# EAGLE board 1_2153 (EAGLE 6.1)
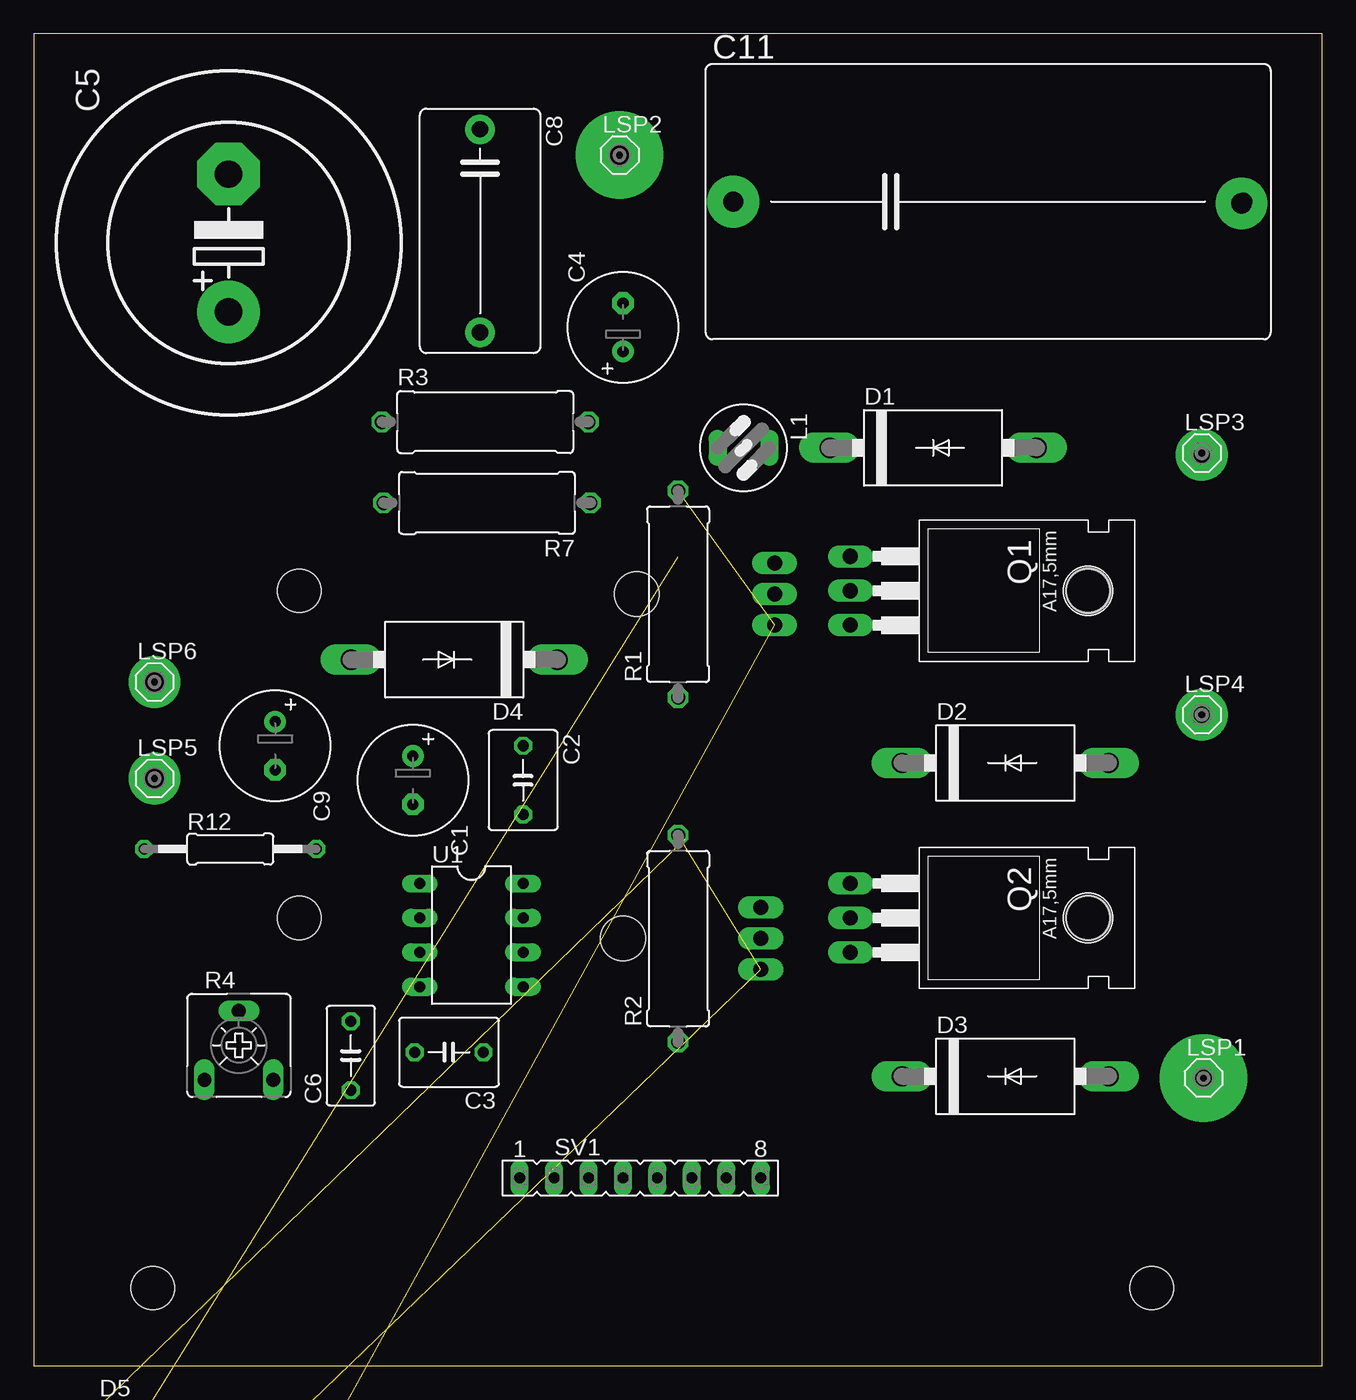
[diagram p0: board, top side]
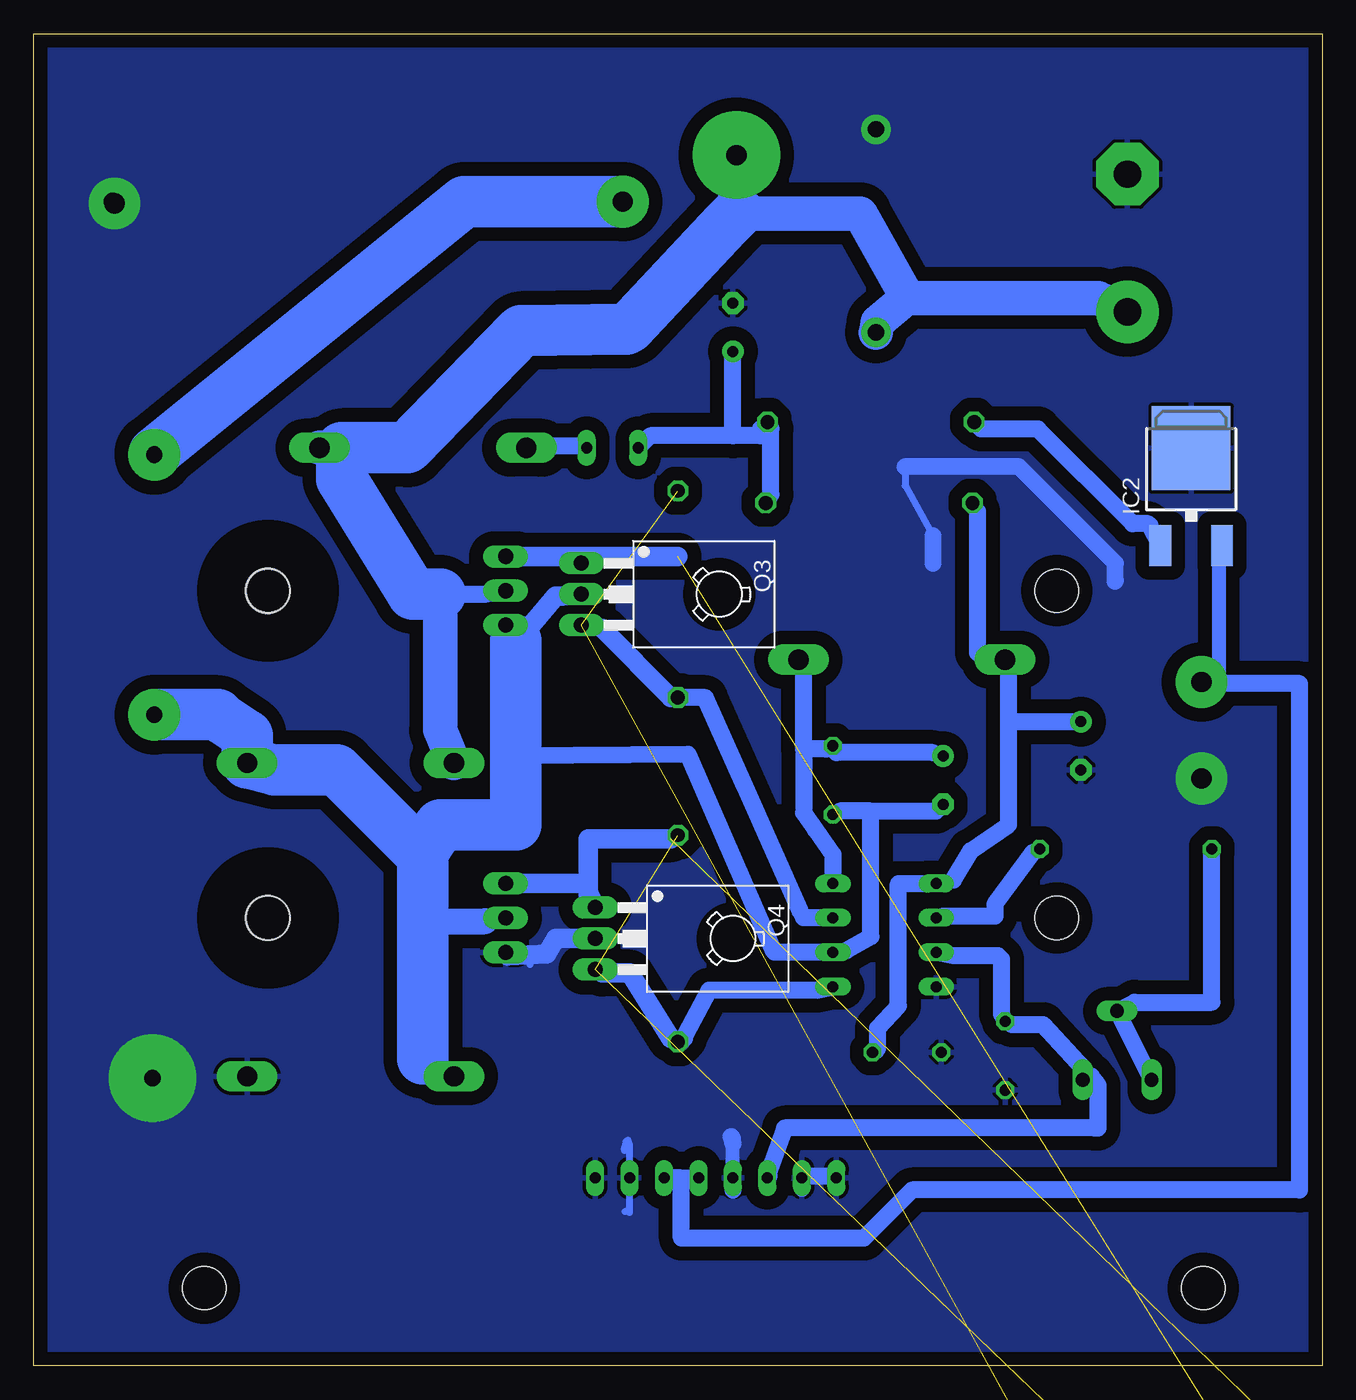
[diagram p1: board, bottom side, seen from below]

Size 94.98 x 98.22 mm. Coordinates in mm from the lower left corner, seen from the top.
Outline: 0,0 94.98,0 94.98,98.22 0,98.22 0,0
Copper layers (1*16): Top 0.035mm / dielectric 1.5mm / Bottom 0.035mm
Design rules: minimum track width 20mil, minimum drill 24mil, track to track 10mil, track to pad 15mil, pad to pad 8mil, via to via 8mil, smd to smd 8mil, copper to edge 40mil, drill to drill 8mil, minimum pad ring 10mil, minimum via ring 8mil, stop-mask expansion 4mil, vias tented up to drill 0mil, thermal gap 10mil
Holes 3.2 mm at 19.56,57.15 19.56,33.02 8.76,5.71 82.42,5.71 77.72,57.15 77.72,33.02

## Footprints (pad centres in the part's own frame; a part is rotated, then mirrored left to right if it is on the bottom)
E3,5-8 = drill 0.813 pad 1.6: + -1.778,0 | drill 0.813 pad 1.6 octagon: - 1.778,0
C050-050X075 = drill 0.813 octagon: 1 -2.54,0; 2 2.54,0
EB25D = drill 2.007 pad 4.597: + -5.08,0 | drill 2.007 pad 4.597 octagon: - 5.08,0
C050-035X075 = drill 0.813 octagon: 1 -2.54,0; 2 2.54,0
C150-091X182 = drill 1.016 octagon: 1 -7.493,0; 2 7.493,0
C375-203X418 = drill 1.321 octagon: 1 -18.796,0; 2 18.796,0
DO201-15 = drill 1.499 long: A 7.62,0; C -7.62,0
DPACK = smd 1.6 x 3: 1 -2.28,-4.8; 3 2.28,-4.8 | smd 5.8 x 6.2: 4 0,2.38
82114R = drill 0.813 long: 1 0,1.905; 2 0,-1.905
MCS10B = drill 1.016 pad 2.159 octagon: MP 0,0
TO220 = drill 1.118 long: 1 -2.54,-6.35; 2 0,-6.35; 3 2.54,-6.35 | hole 3.302: 0,11.176
TO126 = drill 1.118 long: 1 -2.286,-5.08; 2 0,-5.08; 3 2.286,-5.08 | hole 3.302: 0,5.08
P0613/15 = drill 1.016 octagon: 1 -7.62,0; 2 7.62,0
CA6V = drill 1.016 long: A -2.54,-2.54; E 2.54,-2.54; S 0,2.54
0207/12 = drill 0.813 octagon: 1 -6.35,0; 2 6.35,0
FE08 = drill 0.813 long: 1 -8.89,0; 2 -6.35,0; 3 -3.81,0; 4 -1.27,0; 5 1.27,0; 6 3.81,0; 7 6.35,0; 8 8.89,0
DIL08 = drill 0.813 long: 1 -3.81,-3.81; 2 -1.27,-3.81; 3 1.27,-3.81; 4 3.81,-3.81; 5 3.81,3.81; 6 1.27,3.81; 7 -1.27,3.81; 8 -3.81,3.81

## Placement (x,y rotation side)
C1  100x16  [E3,5-8]  27.94,43.18 270 top
C2  0.33  [C050-050X075]  36.07,43.18 270 top
C3  0.33  [C050-050X075]  30.61,23.11 180 top
C4  100x16  [E3,5-8]  43.43,76.58 90 top
C5  [EB25D]  14.35,82.8 90 top
C6  2.2n  [C050-035X075]  23.37,22.86 90 top
C8  2.0  [C150-091X182]  32.89,83.69 270 top
C9  100x35  [E3,5-8]  17.78,45.72 270 top
C11  [C375-203X418]  70.36,85.85 0 top
D1  1N5400  [DO201-15]  66.29,67.69 0 top
D2  1N5400  [DO201-15]  71.63,44.45 0 top
D3  1N5400  [DO201-15]  71.63,21.34 0 top
D4  1N5400  [DO201-15]  30.99,52.07 180 top
D5  1N5400  [DO201-15]  not placed on the board
D6  1N5400  [DO201-15]  not placed on the board
IC2  7812  [DPACK]  9.65,65.28 0 bottom
L1  100mkGn  [82114R]  52.32,67.69 270 top
LSP1  MCS10B  [MCS10B]  86.23,21.21 0 top
LSP2  MCS10B  [MCS10B]  43.18,89.28 0 top
LSP3  MCS10B  [MCS10B]  86.11,67.31 0 top
LSP4  MCS10B  [MCS10B]  86.11,48.01 0 top
LSP5  MCS10B  [MCS10B]  8.89,43.31 0 top
LSP6  MCS10B  [MCS10B]  8.89,50.42 0 top
Q1  IRL3705  [TO220]  66.55,57.15 270 top
Q2  IRL3705  [TO220]  66.55,33.02 270 top
Q3  [TO126]  49.53,56.9 270 bottom
Q4  BD140  [TO126]  48.51,31.5 270 bottom
R1  100  [P0613/15]  47.5,56.9 90 top
R2  100  [P0613/15]  47.5,31.5 90 top
R3  100E  [P0613/15]  33.27,69.6 0 top
R4  10k  [CA6V]  15.11,23.62 0 top
R7  240E  [P0613/15]  33.4,63.63 180 top
R12  1k  [0207/12]  14.48,38.1 0 top
SV1  [FE08]  44.7,13.84 0 top
U1  IR2153  [DIL08]  32.26,31.75 270 top

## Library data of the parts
C1-C6 C8 C9 C11 R1-R3 R7 R12 = rcl
D1-D6 = diode
IC2 = v-reg
L1 = inductors
LSP1-LSP6 = solpad
Q1 Q2 = transistor-fet
Q3 Q4 = transistor-pnp
R4 = pot
SV1 = con-lsta
U1 = irf

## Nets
COM: C6.2 R4.E SV1.3 U1.3
GND: C3.2 C4.- C5.- C6.1 C8.1 C9.- C11.2 D3.A IC2.4 LSP1.MP LSP5.MP Q2.3 Q4.2 SV1.1 SV1.2 SV1.4 SV1.7 SV1.8 U1.4
N$1: D6.A Q3.3 R1.2
N$2: R12.2 U1.2
N$3: D5.A Q4.3 R2.2
N$4: C4.+ L1.2 R3.2 R7.1
N$5: R1.1 U1.7
N$6: R4.A R4.S R12.1
N$7: IC2.3 LSP6.MP SV1.5 SV1.6
N$8: R2.1 U1.5
N$9: IC2.1 R3.1
N$10: D5.C Q2.1 Q4.1
N$11: D6.C Q1.1 Q3.1
N$13: D1.C L1.1
N$19: C11.1 LSP3.MP
N$22: C5.+ C8.2 D1.A D2.C LSP2.MP Q1.2
VB: C1.+ C2.1 D4.C U1.8
VCC: C3.1 C9.+ D4.A R7.2 U1.1
VS: C1.- C2.2 D2.A D3.C LSP4.MP Q1.3 Q2.2 Q3.2 U1.6

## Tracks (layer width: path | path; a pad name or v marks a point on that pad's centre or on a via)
COM
  Bottom 0.508: 23.62,29.97 23.88,30.23 | 16.51,17.53 16.76,17.53 | 40.77,13.97 SV1.3 | 22.86,25.15 C6.2 | R4.E 17.53,21.84
  Bottom 1.27: 23.88,30.23 27.18,30.23 U1.3 | 23.62,29.97 23.62,25.91 C6.2 | 40.77,13.97 40.89,13.97 39.62,17.53 16.76,17.53 | 16.51,17.53 16.51,20.7 17.02,21.34 R4.E | 22.86,25.15 20.57,25.15 17.53,21.84
GND  (via drill 1.2 pad 2.18, 1.2 pad 6.45, 1.5 pad 3.81)
  Bottom 0.508: 57.15,30.35 57.08,30.21 | 60.05,30.23 Q2.3 | 37.85,13.97 SV1.2 | 28.7,60.2 28.78,60.2 | 30.73,66.29 30.73,64.9 28.7,61.21 | 51.05,16.26 51.44,15.88 51.31,16.38 51.18,16.64 51.05,16.26 | 51.05,16.26 51.31,16 51.31,16.51 51.05,16.26 | 51.05,16.26 SV1.7 51.05,11.3 51.4,11.38 | 43.43,16.76 43.56,16.89 | 58.45,30.3 58.42,29.72 58.38,29.57
  Bottom 1.016: SV1.4 43.43,16.38 | 43.48,16.76 43.43,16.76 | SV1.2 38.35,12.95
  Bottom 1.27: 28.7,59.18 28.7,60.2 28.7,61.21 | 43.43,16.38 43.48,16.76 | 37.85,13.97 36.32,13.97 SV1.1 | 30.73,66.29 22.35,66.29 15.24,59.18 15.24,57.91 15.25,57.85 | 43.56,16.89 43.55,16.9 | SV1.4 43.43,12.95
  Bottom 1.422: Q4.2 56.52,31.5 57.15,30.35 58.45,30.3 60.05,30.23
  other vias: 8.89,43.31 86.23,21.21 32.89,91.19 89.03,85.72
  pour Bottom (isolate 1.016): 0,-0.25 0.38,98.04 94.87,98.17 95,94.87 95,83.95 94.87,75.56 95.12,65.91 94.87,30.1 95.12,-0.13
LSP2  (via drill 1.5 pad 6.45)
  other vias: 43.18,89.28
LSP6  (via drill 1.5 pad 3.81)
  other vias: 8.89,50.42
N$1  (2 unrouted)
N$2
  Bottom 0.508: 27.94,33.15 28.32,33.02
  Bottom 1.27: 27.94,33.15 24.13,33.15 24.13,34.04 21.34,37.85 R12.2 | 28.32,33.02 U1.2
N$3  (2 unrouted)
N$4
  Bottom 0.508: R3.2 41.4,69.09
  Bottom 1.27: 43.43,68.58 41.4,68.58 41.4,69.09 | 43.43,68.58 49.53,68.58 L1.2 | R7.1 40.64,64.26 40.64,69.09 R3.2 | 43.43,68.58 C4.+
N$5
  Bottom 1.27: U1.7 38.23,33.02 38.48,33.53 42.55,42.67 45.47,49.28 R1.1
  Bottom 1.422: 53.09,54.36 48.01,49.28 R1.1
N$6
  Bottom 1.27: R12.1 8.13,26.8 13.84,26.8 R4.S R4.A
N$7
  Bottom 0.508: 33.78,9.4 34.04,9.4 | 7.62,50.29 IC2.3
  Bottom 1.016: LSP6.MP 7.62,50.42 7.62,59.18 IC2.3
  Bottom 1.27: 7.62,50.29 1.65,50.29 1.65,12.95 30.23,12.95 33.78,9.4 | 34.04,9.4 47.24,9.4 47.24,13.84 | 47.24,13.84 SV1.6 | 47.24,13.84 SV1.5
N$8
  Bottom 1.27: U1.5 37.34,27.69 45.21,27.69 47.24,23.88 46.99,24.13 R2.1 48.01,24.13
  Bottom 1.422: 53.09,28.96 51.05,28.96 48.01,24.13
N$9
  Bottom 0.508: 12.7,61.98 12.83,62.1
  Bottom 1.27: 12.83,62.1 13.97,62.1 20.95,69.09 25.15,69.09 R3.1 | IC2.1 12.7,61.98
N$10  (1 unrouted)
  Bottom 0.508: Q4.1 54.1,34.54
  Bottom 1.422: 48.01,38.86 54.1,38.86 54.1,34.54 | Q2.1 54.36,35.56 Q4.1
N$11  (1 unrouted)
  Bottom 1.422: 47.5,59.69 54.61,59.69 | 54.61,59.69 Q1.1 | 54.61,59.69 Q3.1
N$13
  Bottom 1.27: L1.1 54.61,67.82 56.64,67.82 D1.C
N$14  (via drill 1.2 pad 2.18)
  other vias: 32.89,76.2
N$19  (via drill 1.5 pad 3.81)
  Bottom 3.81: C11.1 63.25,85.85 LSP3.MP
  other vias: 51.56,85.85
N$22
  Bottom 0.508: 30.48,78.74 30.67,78.93 | 43.31,84.96 43.05,85.09
  Bottom 1.27: 65.02,56.9 61.72,56.9 Q1.2 | 30.67,78.93 30.48,78.87
  Bottom 2.54: 65.02,56.9 65.02,46.86 D2.C | 72.26,67.69 D1.A | 30.48,78.74 16.51,78.74 C5.+ | 30.67,78.93 34.04,84.96 43.31,84.96 LSP2.MP | C8.2 32.77,76.96 30.48,78.87
  Bottom 3.81: 65.02,56.9 67.06,56.9 72.26,65.41 72.26,67.69 67.44,67.69 59.05,76.33 51.31,76.45 51.05,76.58 43.94,84.2 43.05,85.09
N$31  (via drill 1.2 pad 3.81)
  other vias: 86.11,67.18
N$32  (via drill 1.2 pad 3.81)
  other vias: 86.11,48.01
VB
  Bottom 0.508: 36.58,45.47 C2.1 35.81,45.21 | C1.+ 28.7,45.21
  Bottom 1.27: 38.23,45.47 38.23,40.77 37.34,39.5 36.07,37.72 U1.8 | 36.58,45.47 38.23,45.47 | 28.7,45.21 35.81,45.21 | 38.23,45.47 38.23,51.05 D4.C
VCC
  Bottom 0.508: 27.18,35.81 U1.1 29.21,35.56 | D4.A 24.64,52.83
  Bottom 1.27: 27.18,35.81 25.91,37.97 23.11,39.88 23.11,47.5 | 23.11,47.5 23.11,51.05 D4.A 25.4,52.58 25.4,62.99 R7.2 | 29.21,35.56 31.24,35.56 31.24,26.54 32.77,24.89 32.77,23.37 32.89,23.24 C3.1 | 23.11,47.5 C9.+
VS
  Bottom 0.508: 61.72,32.77 Q2.2 | 66.29,22.61 D3.C | 66.42,37.72 66.29,37.59 | 35.56,40.89 C2.2 | 28.45,40.89 C1.- | 58.29,54.61 Q1.3 59.44,53.47 | 35.05,30.61 U1.6
  Bottom 1.27: U1.6 40.39,30.48 46.74,45.09 59.44,44.96 | 33.27,40.89 28.45,40.89 | 33.27,40.89 35.56,40.89 | 33.27,40.89 33.27,31.62 35.05,30.61
  Bottom 1.422: 58.29,54.61 56.52,56.77 56.01,56.77 Q3.2
  Bottom 1.93: 66.29,32.77 61.72,32.77
  Bottom 2.54: 81.15,47.75 81.41,48.01 | 66.29,33.02 66.29,32.77
  Bottom 3.81: 81.15,47.75 79.25,46.48 D2.A 77.22,43.94 72.64,43.94 66.42,37.72 65.02,39.88 59.44,39.88 59.44,44.96 59.44,53.47 | 81.41,48.01 LSP4.MP | 66.29,32.77 66.29,22.61 | 66.29,37.59 66.29,33.02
